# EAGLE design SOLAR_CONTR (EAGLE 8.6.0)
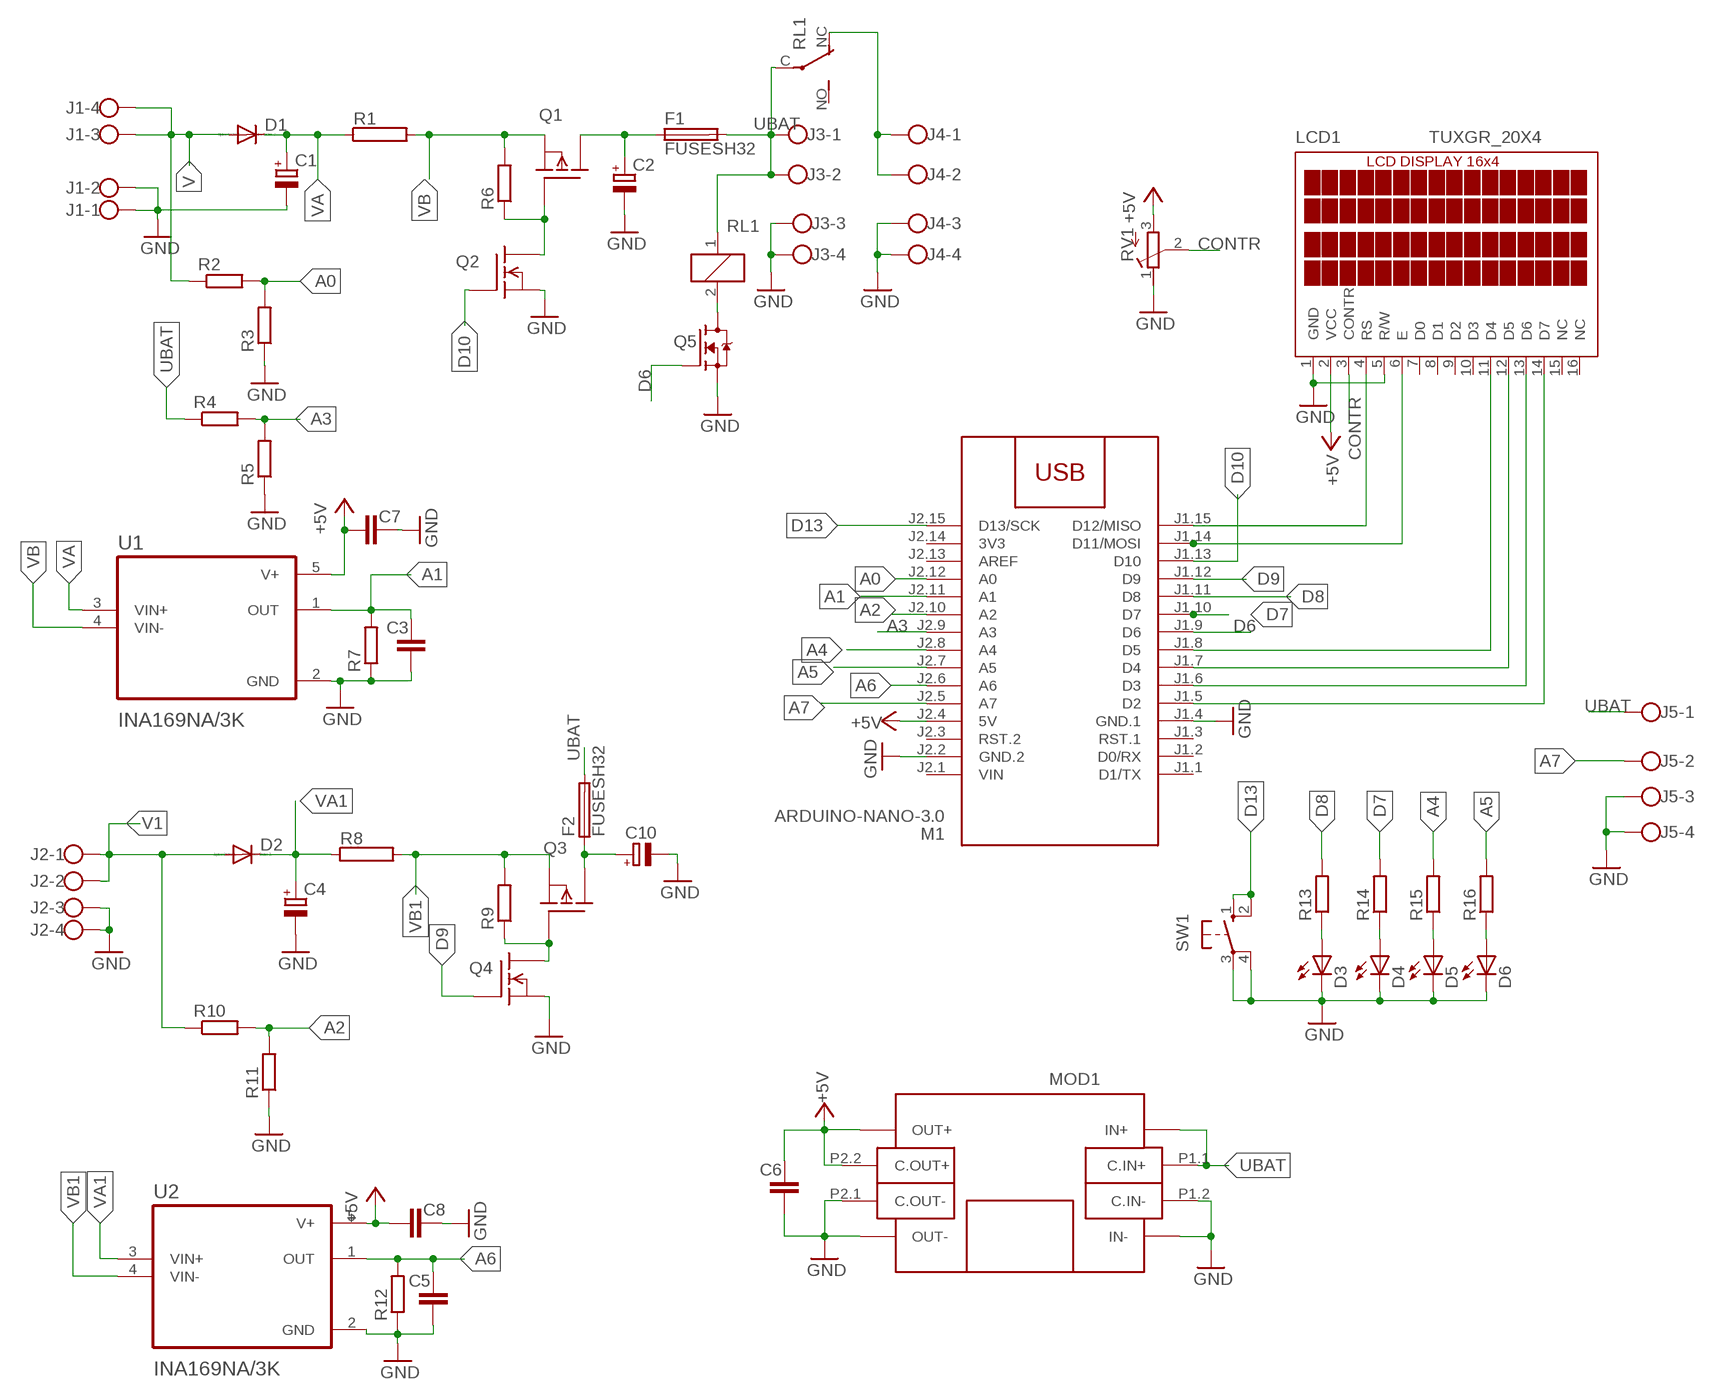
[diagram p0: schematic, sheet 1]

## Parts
C1  CPOL-EUE7.5-16  [E7,5-16]
C2  CPOL-EUE7.5-16  [E7,5-16]
C3  C-EUC1206  [C1206]
C4  CPOL-EUE7.5-16  [E7,5-16]
C5  C-EUC1206  [C1206]
C6  C-EUC1206  [C1206]
C7  C-EUC1206  [C1206]
C8  C-EUC1206  [C1206]
C10  CPOL-EUE7.5-16  [E7,5-16]
D1  BYT08P  [TO220ACS]
D2  BYT08P  [TO220ACS]
D3  LED5MM  [LED5MM]
D4  LED5MM  [LED5MM]
D5  LED5MM  [LED5MM]
D6  LED5MM  [LED5MM]
F1  FUSESH32  [SH32]
F2  FUSESH32  [SH32]
J1  W237-4  [W237-4]
J2  W237-4  [W237-4]
J3  W237-4  [W237-4]
J4  W237-4  [W237-4]
J5  W237-4  [W237-4]
LCD1  TUXGR_20X4  [TUXGR_20X4]
M1  ARDUINO-NANO-3.0  [ARDUINO-NANO-3.0]
MOD1  DC-DC-LM2596-DISP#RC  [DC-DC-LM2596-DISP#RC]
Q1  BUZ171  [TO220]
Q2  VN2222KM  [TO237]
Q3  BUZ171  [TO220]
Q4  VN2222KM  [TO237]
Q5  NTF3055L108  [SOT223]
R1  RAC05  [AC05]
R2  R-EU_R1206  [R1206]
R3  R-EU_R1206  [R1206]
R4  R-EU_R1206  [R1206]
R5  R-EU_R1206  [R1206]
R6  R-EU_R1206  [R1206]
R7  R-EU_R1206  [R1206]
R8  RAC05  [AC05]
R9  R-EU_R1206  [R1206]
R10  R-EU_R1206  [R1206]
R11  R-EU_R1206  [R1206]
R12  R-EU_R1206  [R1206]
R13  R-EU_R1206  [R1206]
R14  R-EU_R1206  [R1206]
R15  R-EU_R1206  [R1206]
R16  R-EU_R1206  [R1206]
RL1  JTN-PCB-DC9V  [JT-PCB]
RV1  R-TRIMM-3386-F  [R-TRIMM-3386F]
SW1  40-XX  [B3F-40XX]
U1  INA169NA/3K  [SOT95P280X145-5N]
U2  INA169NA/3K  [SOT95P280X145-5N]

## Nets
+5V: C6.1 C7.1 C8.1 LCD1.2(VCC) M1.J2.4(5V) MOD1.OUT+ MOD1.P2.2(C.OUT+) RV1.3(E) U1.5(V+) U2.5(V+)
A0: M1.J2.12(A0) R2.2 R3.2
A1: C3.1 M1.J2.11(A1) R7.2 U1.1(OUT)
A2: M1.J2.10(A2) R10.2 R11.2
A3: M1.J2.9(A3) R4.2 R5.2
A4: M1.J2.8(A4) R15.2
A5: M1.J2.7(A5) R16.2
A6: C5.1 M1.J2.6(A6) R12.2 U2.1(OUT)
A7: J5.2 M1.J2.5(A7)
CONTR: LCD1.3(CONTR) RV1.2(S)
D6: M1.J1.9(D6) Q5.1(G)
D7: M1.J1.10(D7) R14.2
D8: M1.J1.11(D8) R13.2
D9: M1.J1.12(D9) Q4.2(G)
D10: M1.J1.13(D10) Q2.2(G)
D13: M1.J2.15(D13/SCK) SW1.1(S) SW1.2(S1)
GND: C1.- C2.- C3.2 C4.- C5.2 C6.2 C7.2 C8.2 C10.- D3.K(C) D4.K(C) D5.K(C) D6.K(C) J1.1 J1.2 J2.3 J2.4 J3.3 J3.4 J4.3 J4.4 J5.3 J5.4 LCD1.1(GND) LCD1.5(R/W) M1.J1.4(GND.1) M1.J2.2(GND.2) MOD1.IN- MOD1.OUT- MOD1.P1.2(C.IN-) MOD1.P2.1(C.OUT-) Q2.3(S) Q4.3(S) Q5.3(S) R3.1 R5.1 R7.1 R11.1 R12.1 RV1.1(A) SW1.3(P) SW1.4(P1) U1.2(GND) U2.2(GND)
N$1: LCD1.4(RS) M1.J1.15(D12/MISO)
N$2: LCD1.6(E) M1.J1.14(D11/MOSI)
N$3: LCD1.11(D4) M1.J1.8(D5)
N$4: LCD1.12(D5) M1.J1.7(D4)
N$5: LCD1.13(D6) M1.J1.6(D3)
N$6: LCD1.14(D7) M1.J1.5(D2)
N$7: C2.+ F1.1A Q1.2(D)
N$8: Q5.2(D) Q5.4(D) RL1.2
N$9: Q1.1(G) Q2.1(D) R6.1
N$10: Q3.1(G) Q4.1(D) R9.1
N$11: C10.+ F2.1A Q3.2(D)
N$13: J4.1 J4.2 RL1.NC(O)
N$14: D3.A R13.1
N$15: D4.A R14.1
N$16: D5.A R15.1
N$17: D6.A R16.1
UBAT: F1.2A F2.2A J3.1 J3.2 J5.1 MOD1.IN+ MOD1.P1.1(C.IN+) R4.1 RL1.1 RL1.C(P)
V: D1.A J1.3 J1.4 R2.1
V1: D2.A J2.1 J2.2 R10.1
VA: C1.+ D1.C R1.1 U1.3(VIN+)
VA1: C4.+ D2.C R8.1 U2.3(VIN+)
VB: Q1.3(S) R1.2 R6.2 U1.4(VIN-)
VB1: Q3.3(S) R8.2 R9.2 U2.4(VIN-)
Unconnected: LCD1.7(D0) LCD1.8(D1) LCD1.9(D2) LCD1.10(D3) LCD1.15(NC) LCD1.16(NC) M1.J1.1(D1/TX) M1.J1.2(D0/RX) M1.J1.3(RST.1) M1.J2.3(RST.2) M1.J2.13(AREF) RL1.NO(S)

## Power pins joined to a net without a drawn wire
3V3: M1.J2.14(3V3)
VIN: M1.J2.1(VIN)

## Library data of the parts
C1 C2 C4 C10 = rcl:CPOL-EU: POLARIZED CAPACITOR, European symbol
C3 C5-C8 = rcl:C-EU: CAPACITOR, European symbol
D1 D2 = diode:BYT08P: DIODE
D3-D6 = led:LED: LED
F1 F2 = fuse:FUSE: Fuse; OC_FARNELL: unknown; OC_NEWARK: unknown
J1-J5 = con-wago-500:W237-4: WAGO SCREW CLAMP; OC_FARNELL: unknown; OC_NEWARK: unknown
LCD1 = display-lcd:TUXGR_20X4: LCD DISPLAY 20X4
M1 = diy-modules:ARDUINO-NANO-3.0: Arduino Nano 3.0 and compatible devices More details available here: https://www.arduino.cc/en/Main/ArduinoBoardNano Click here to find device on ebay.com
MOD1 = diy-modules:DC-DC-LM2596-DISP#RC: DC/DC Step-Down Regulator with Voltage Display based on LM2596-ADJ chip Symbol with input and output connectors More details available here: http://www.instructables.com/id/The-Introduction-of-LM2596-Step-Down-Power-Module-/ LM2596 datasheet available here: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
Q1 Q3 = transistor-fet:BUZ171: P-Channel Enhancement MOSFET -50V; 7A; 0,4Ohm
Q2 Q4 = transistor-fet:VN2222KM: N-Channel Enhancement MOSFET (VMOS); 60V; 0,5A; 7,5Ohm
Q5 = transistor-fet:NTF3055L108
R1 R8 = resistor-power:R: Power Resitor; OC_FARNELL: unknown; OC_NEWARK: unknown
R2-R7 R9-R16 = rcl:R-EU_: RESISTOR, European symbol
RL1 = relay:JT?-*: COMPACT ECONOMICAL 30 AMP. RELAY NAiS Source: http://www.mew-europe.com/.. en_ds_61212_0000.pdf; OC_FARNELL: unknown; OC_NEWARK: unknown
RV1 = rcl:R-TRIMM-3386-F
SW1 = switch-omron:40-XX: OMRON SWITCH; MF: OMRON COMPONENTS USA; MPN: B3F-4000; OC_FARNELL: 176434; OC_NEWARK: 36K3105
U1 U2 = INA169NA_3K:INA169NA/3K: Check availability; AVAILABILITY: In Stock; CHECK_PRICES: https://www.snapeda.com/parts/INA169NA/3K/Texas+Instruments/view-part/?ref=eda; DESCRIPTION: 2.7 to 60V, 440kHz Variable gain current sense amplifier; MF: Texas Instruments; MP: INA169NA/3K; PACKAGE: SOT-23-5 Texas Instruments; PRICE: None; PURCHASE-URL: https://pricing.snapeda.com/search?q=INA169NA/3K&ref=eda; SNAPEDA_LINK: https://www.snapeda.com/parts/INA169NA/3K/Texas+Instruments/view-part/?ref=snap

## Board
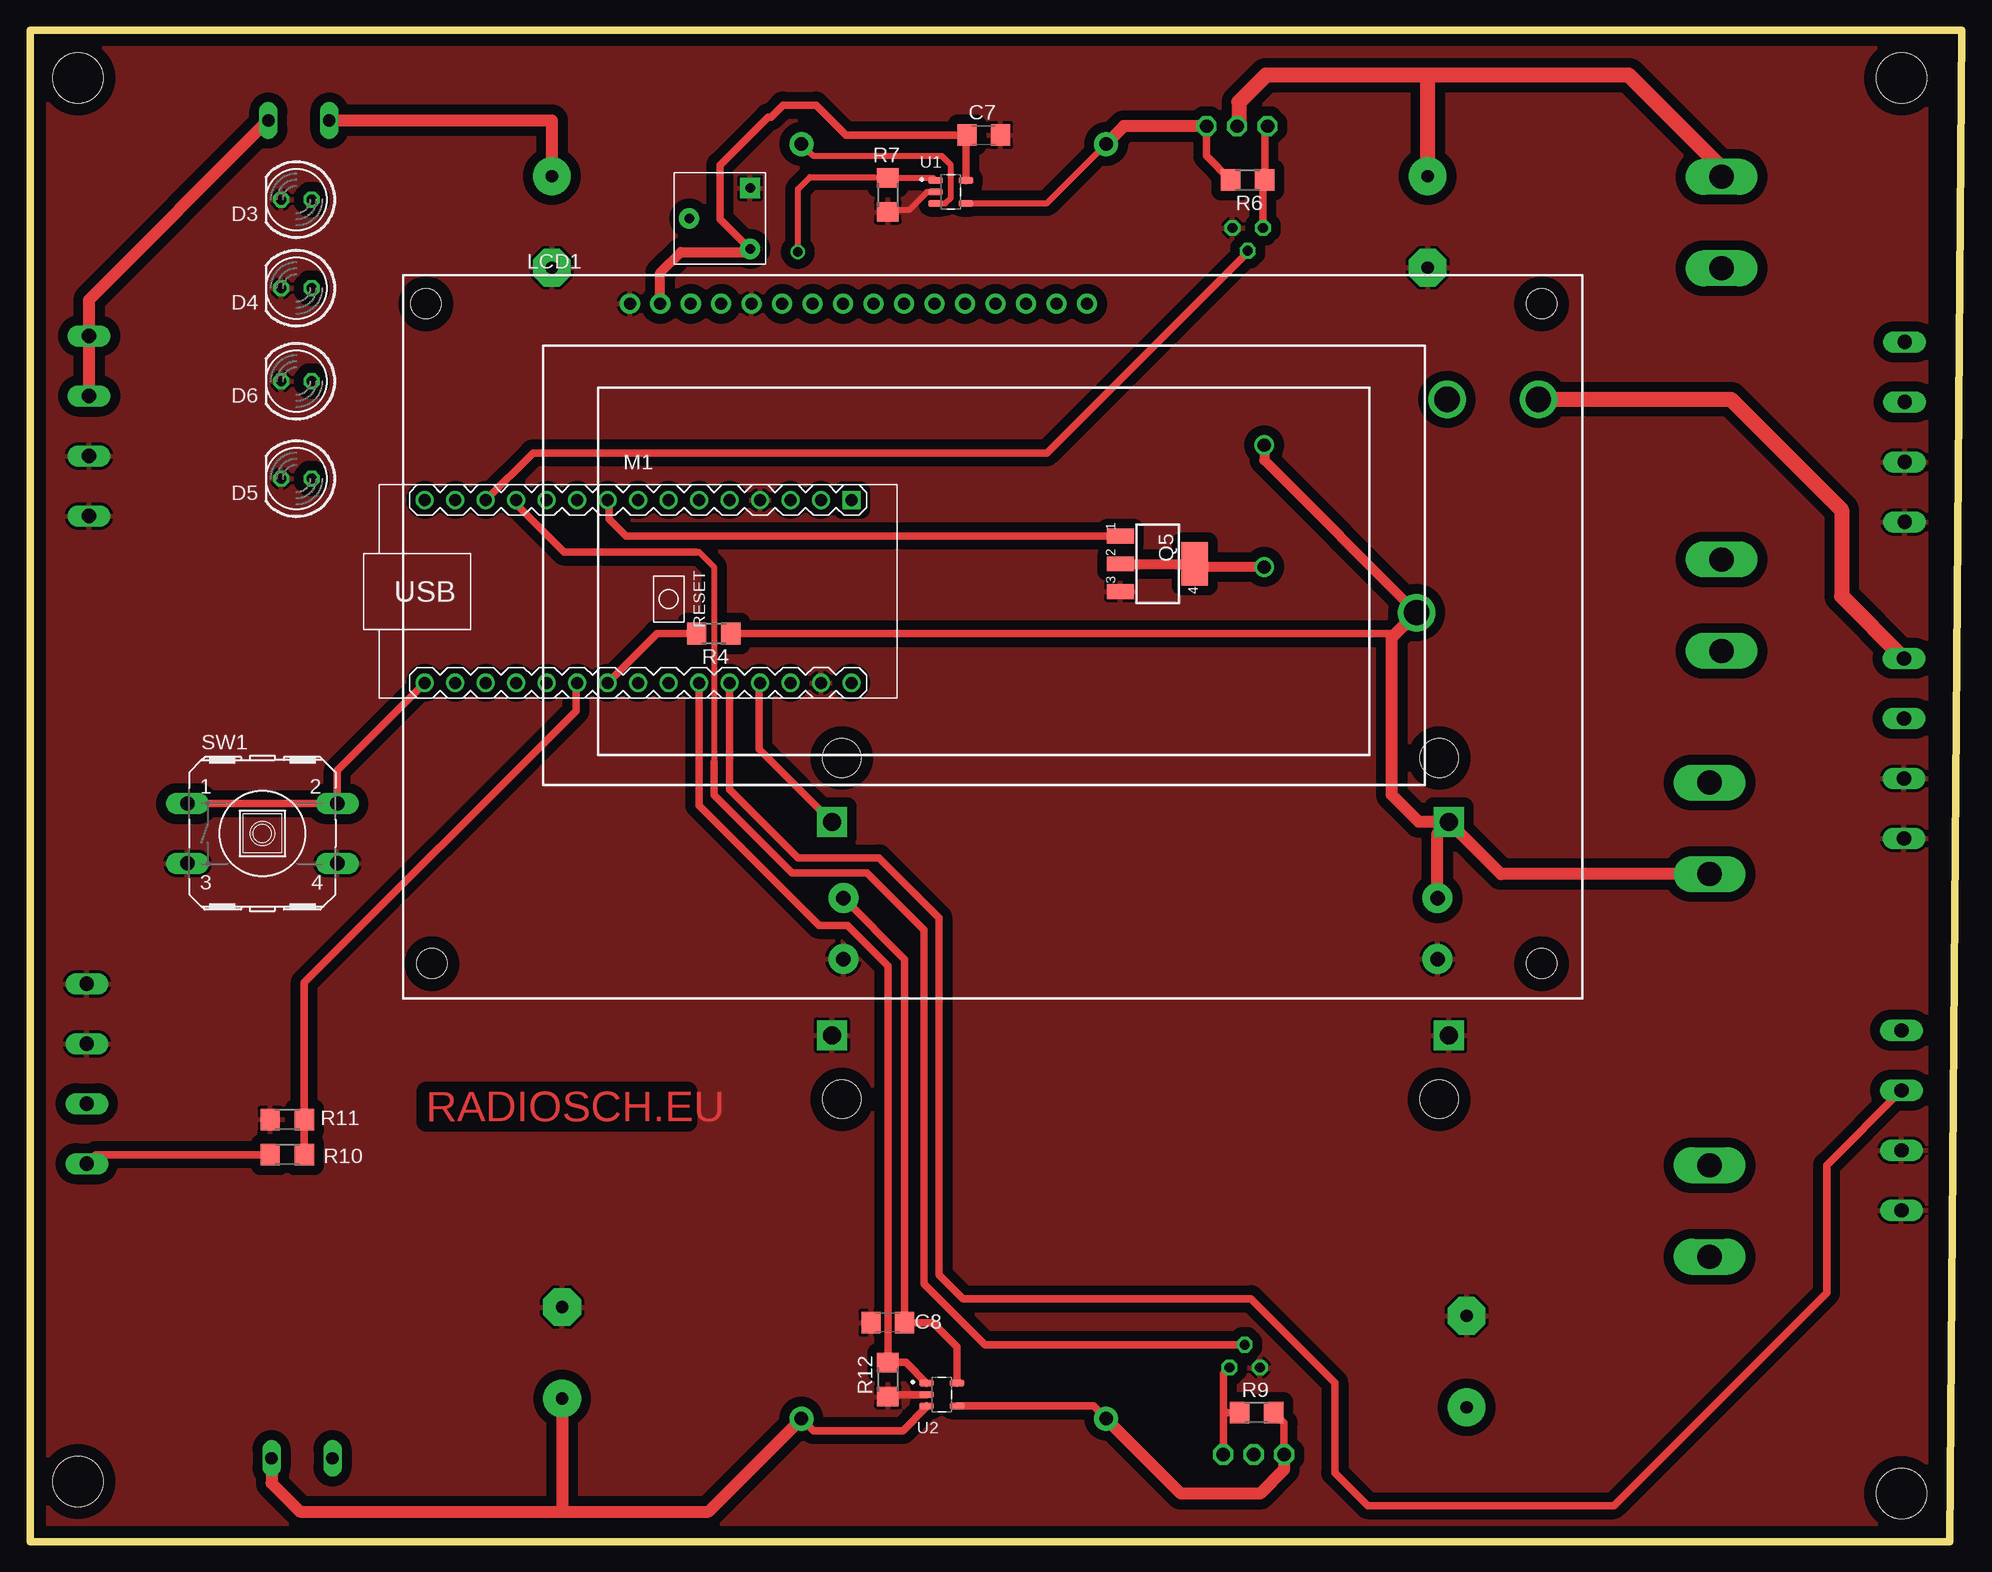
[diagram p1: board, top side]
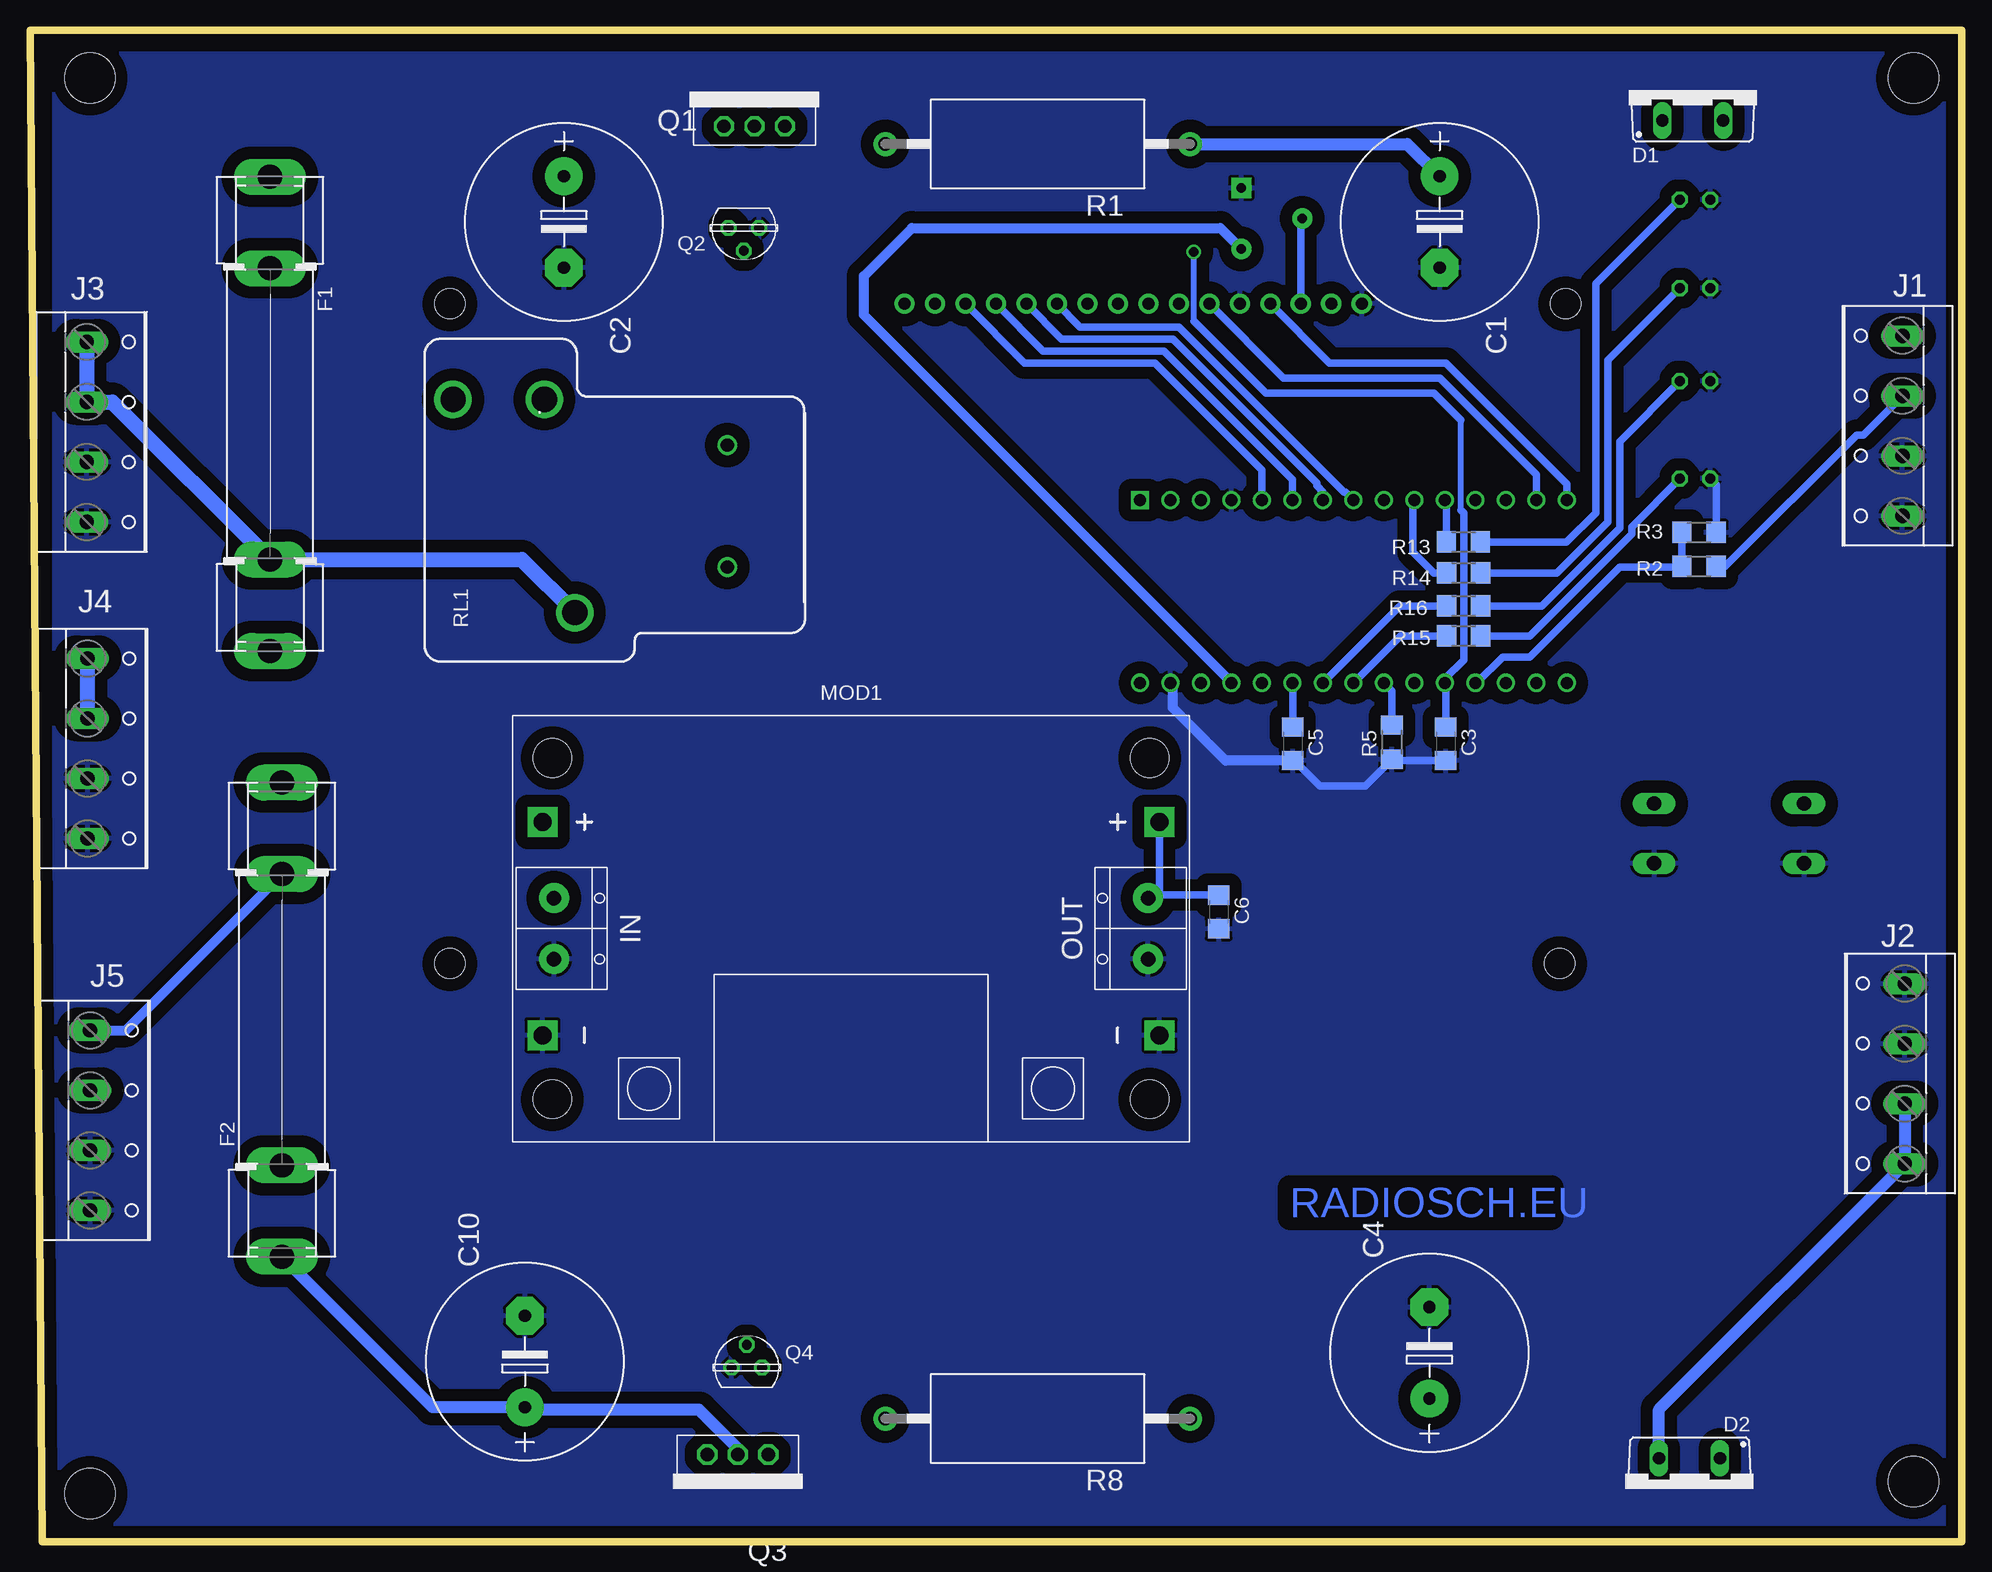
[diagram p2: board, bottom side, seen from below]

Size 161 x 126 mm. Coordinates in mm from the lower left corner, seen from the top.
Outline: 0,0 160,0 161,126 0,126 0,0
Copper layers (1*16): Top 0.035mm / dielectric 1.5mm / Bottom 0.035mm
Design rules "default": minimum track width 10mil, minimum drill 24mil, track to track 8mil, track to pad 8mil, pad to pad 8mil, via to via 8mil, smd to smd 8mil, copper to edge 40mil, drill to drill 8mil, minimum pad ring 10mil, minimum via ring 8mil, stop-mask expansion 4mil, vias tented up to drill 0mil, thermal gap 10mil
Holes 4.2 mm at 4,122 4,5 156,4 156,122

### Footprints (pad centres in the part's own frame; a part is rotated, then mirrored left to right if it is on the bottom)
E7,5-16 = drill 1.016 pad 3.15: + -3.81,0 | drill 1.016 pad 3.15 octagon: - 3.81,0
C1206 = smd 1.6 x 1.8: 1 -1.4,0; 2 1.4,0
TO220ACS = drill 1.016 long: A 2.54,-2.54; C -2.54,-2.54
LED5MM = drill 0.813 octagon: A -1.27,0; K 1.27,0
SH32 = drill 2.007 long: 1A -16.764,0; 1B -9.144,0; 2A 15.144,0; 2B 22.764,0
W237-4 = drill 1.194 long: 1 -7.5,-1.27; 2 -2.5,-1.27; 3 2.5,-1.27; 4 7.5,-1.27
TUXGR_20X4 = drill 1 pad 1.676: 1 11.14,-2.28; 2 13.68,-2.28; 3 16.22,-2.28; 4 18.76,-2.28; 5 21.3,-2.28; 6 23.84,-2.28; 7 26.38,-2.28; 8 28.92,-2.28; 9 31.46,-2.28; 10 34,-2.28; 11 36.54,-2.28; 12 39.08,-2.28; 13 41.62,-2.28; 14 44.16,-2.28; 15 46.7,-2.28; 16 49.24,-2.28 | hole 2.5: -5.36,-57.28; 87.14,-57.28; -5.86,-2.28; 87.14,-2.28
ARDUINO-NANO-3.0 = drill 1 square: J1.1 17.78,7.62 | drill 1: J1.2 15.24,7.62; J1.3 12.7,7.62; J1.4 10.16,7.62; J1.5 7.62,7.62; J1.6 5.08,7.62; J1.7 2.54,7.62; J1.8 0,7.62; J1.9 -2.54,7.62; J1.10 -5.08,7.62; J1.11 -7.62,7.62; J1.12 -10.16,7.62; J1.13 -12.7,7.62; J1.14 -15.24,7.62; J1.15 -17.78,7.62; J2.1 17.78,-7.62; J2.2 15.24,-7.62; J2.3 12.7,-7.62; J2.4 10.16,-7.62; J2.5 7.62,-7.62; J2.6 5.08,-7.62; J2.7 2.54,-7.62; J2.8 0,-7.62; J2.9 -2.54,-7.62; J2.10 -5.08,-7.62; J2.11 -7.62,-7.62; J2.12 -10.16,-7.62; J2.13 -12.7,-7.62; J2.14 -15.24,-7.62; J2.15 -17.78,-7.62
DC-DC-LM2596-DISP#RC = drill 1.5 pad 2.5 square: IN+ -25.718,8.89; IN- -25.718,-8.89; OUT+ 25.718,8.89; OUT- 25.718,-8.89 | drill 1.2 pad 2.5: P1.1 -24.765,2.54; P1.2 -24.765,-2.54; P2.1 24.765,-2.54; P2.2 24.765,2.54 | hole 3.2: -24.892,14.224; 24.892,-14.224; 24.892,14.224; -24.892,-14.224
TO220 = drill 1.118 octagon: 1 -2.54,0; 2 0,0; 3 2.54,0
TO237 = drill 0.813 octagon: 1 1.27,0; 2 0,1.905; 3 -1.27,0
SOT223 = smd 1.219 x 2.235: 1 -2.311,-3.099; 2 0,-3.099; 3 2.311,-3.099 | smd 3.6 x 2.2: 4 0,3.099
AC05 = drill 1.1 pad 2: 1 -12.7,0; 2 12.7,0
R1206 = smd 1.6 x 1.803: 1 -1.422,0; 2 1.422,0
JT-PCB = drill 1.1: 1 5.08,0; 2 -5.08,0 | drill 2.1: C -8.89,12.7; NC 8.89,22.86; NO 8.89,15.24
R-TRIMM-3386F = drill 0.8 pad 1.676 square: 1 0,0 | drill 0.8 pad 1.676: 2 5.08,2.54; 3 0,5.08
B3F-40XX = drill 1.194 long: 1 -6.248,2.489; 2 6.248,2.489; 3 -6.248,-2.489; 4 6.248,-2.489
SOT95P280X145-5N = smd 1.21 x 0.59: 1 -1.255,0.95; 2 -1.255,0; 3 -1.255,-0.95; 4 1.255,-0.95; 5 1.255,0.95

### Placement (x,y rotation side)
C1  43.5,110 270 bottom
C2  116.5,110 270 bottom
C3  43,66.5 270 bottom
C4  44.35,15.73 90 bottom
C5  55.75,66.5 270 bottom
C6  61.91,52.48 270 bottom
C7  79.5,117.25 0 top
C8  71.5,18.25 180 top
C10  119.75,15 90 bottom
D1  22.41,121 0 bottom
D2  22.67,4.39 180 bottom
D3  22.21,111.86 180 top
D4  22.21,104.48 180 top
D5  22.21,88.6 180 top
D6  22.21,96.72 180 top
F1  141,97 270 bottom
F2  140,40.5 90 bottom
J1  6.2,93 90 bottom
J2  6,39 90 bottom
J3  155,92.5 270 bottom
J4  154.93,66.11 270 bottom
J5  154.72,35.11 270 bottom
LCD1  38.86,105.46 0 top
M1  50.69,79.2 0 top
MOD1  92.56,51.09 0 bottom
Q1  100.61,117.98 0 bottom
Q2  101.5,109.5 180 bottom
Q3  102,7.25 180 bottom
Q4  101.25,14.5 0 bottom
Q5  94,81.5 270 top
R1  77,116.5 180 bottom
R2  21.88,81.28 180 bottom
R3  21.88,84.11 180 bottom
R4  56.99,75.69 180 top
R5  47.48,66.63 90 bottom
R6  101.5,113.5 180 top
R7  71.5,112.25 90 top
R8  77,10.25 180 bottom
R9  102.25,10.75 0 top
R10  21.45,32.25 0 top
R11  21.45,35.17 0 top
R12  71.5,13.5 90 top
R13  41.52,83.32 180 bottom
R14  41.5,80.75 180 bottom
R15  41.5,75.5 180 bottom
R16  41.5,78 180 bottom
RL1  102.88,86.32 90 bottom
RV1  60.03,112.83 180 top
SW1  19.37,59.03 0 top
U1  76.75,112.5 0 top
U2  76,12.25 0 top

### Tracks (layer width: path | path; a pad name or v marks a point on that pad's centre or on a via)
+5V
  Top 0.61: RV1.3 60,107.75 57.5,110.25 57.5,114.75 61.5,118.75 61.75,118.75 62.75,119.75 65.5,119.75 68,117.25 C7.1 78,117.16 U1.5 | M1.J2.4 60.75,71.48 60.75,66.07 MOD1.OUT+ | MOD1.P2.2 72.9,48.52 C8.1 75.25,18.25 77.25,16.25 U2.5
  Top 0.813: LCD1.2 52.54,105.79 54.25,107.5 59.78,107.5 RV1.3
  Bottom 0.61: C6.1 67.25,53.88 | 67.25,53.88 67.55,53.88 MOD1.P2.2 | MOD1.OUT+ 66.84,54.29 67.25,53.88
  Bottom 0.813: M1.J2.4 60.85,71.6 91.5,102.25 91.5,105.5 87.5,109.5 61.78,109.5 RV1.3
A0
  Bottom 0.61: M1.J2.12 40.42,71.58 38.25,73.75 36,73.75 28.5,81.25 23.33,81.25 R2.2 R3.2
A1  (via drill 0.8)
  Top 0.51: U1.1 75.27,113.67 R7.2 71.42,113.75 65,113.75 64,112.75 v64,107.5
  Bottom 0.5: 41.75,86 41.75,93.5 | 64,101.75 v64,107.5
  Bottom 0.61: C3.1 43,71.51 M1.J2.11 43.07,71.93 41.5,73.5 41.5,85.75 41.75,86 | 41.75,93.5 44,95.75 58,95.75 64,101.75
A2
  Top 0.61: R10.2 R11.2 22.87,46.62 45.5,69.25 45.5,71.47 M1.J2.10
A3
  Top 0.61: R4.2 52.26,75.69 M1.J2.9
  Bottom 0.61: R5.2 47.48,70.91 M1.J2.9
A4
  Bottom 0.61: R15.2 46.77,75.5 M1.J2.8
A5
  Bottom 0.61: R16.2 46.81,78 M1.J2.7
A6
  Top 0.61: M1.J2.6 55.75,71.56 55.75,61.38 65.75,51.38 68.12,51.38 71.5,48 R12.2 73.02,14.92 U2.1
  Bottom 0.61: C5.1 55.75,71.56 M1.J2.6
A7
  Top 0.61: M1.J2.5 58.31,62.69 64,57 70.75,57 75.75,52 75.75,22.25 77.75,20.25 101.75,20.25 108.75,13.25 108.75,5.75 111.5,3 132,3 149.75,20.75 149.75,31.37 J5.2
CONTR
  Bottom 0.61: LCD1.3 55.08,110.16 RV1.2
D6
  Top 0.61: Q5.1 49.69,83.81 48.25,85.25 48.25,86.72 M1.J1.9
D7
  Bottom 0.61: R14.2 44,80.75 45.75,82.5 45.75,86.68 M1.J1.10
D8
  Bottom 0.61: R13.2 42.94,86.69 M1.J1.11
D9
  Top 0.51: 55.5,82.5 55.75,82.5 57,81.25 57,65
  Top 0.61: M1.J1.12 40.53,86.47 44.5,82.5 55.5,82.5 | 57,65 57,62.25 63.5,55.75 69.75,55.75 74.5,51 74.5,21.5 79.59,16.41 Q4.2
D10
  Top 0.61: Q2.2 101.5,107.5 84.75,90.75 41.92,90.75 M1.J1.13
D13
  Top 0.61: SW1.1 SW1.2 25.62,64.29 M1.J2.15
GND
  Top 0.51: U1.2 74.75,112.5 73.25,111 71.67,111 R7.1
  Top 0.61: U2.2 71.67,12.25 R12.1
  Bottom 0.61: C3.2 47.37,65.1 R5.1 49.69,63 53.5,63 55.6,65.1 C5.2 | R3.1 20.46,88.12 D5.K
  Bottom 0.813: C5.2 61.35,65.1 65.75,69.5 65.75,71.4 M1.J2.2
  pour Top (isolate 0.813): 1,125 158,125 158,1 1,1
  pour Bottom (isolate 1.016): 159,124 159,1 0.75,1 0.75,124
N$1
  Bottom 0.61: M1.J1.15 32.91,88.16 43,98.25 52.69,98.25 LCD1.4
N$2
  Bottom 0.61: M1.J1.14 35.45,88.95 43.5,97 56.52,97 LCD1.6
N$3
  Bottom 0.61: LCD1.11 73.47,101.25 65.25,101.25 51.5,87.5 51.37,87.5 M1.J1.8
N$4
  Bottom 0.61: M1.J1.7 53.23,87.5 53.75,88.02 53.75,88.25 65.75,100.25 75.01,100.25 LCD1.12
N$5
  Bottom 0.61: M1.J1.6 55.77,88.52 66.5,99.25 76.55,99.25 LCD1.13
N$6
  Bottom 0.61: M1.J1.5 58.31,89.31 67.25,98.25 78.09,98.25 LCD1.14
N$7
  Top 1.27: F1.1A 141,114.5 133.25,122.25 116.5,122.25 | 116.5,122.25 103,122.25 100.75,120 100.75,118.12 Q1.2 | C2.+ 116.5,122.25
N$8
  Top 0.813: Q5.2 96.5,81.5 | 96.5,81.5 Q5.4 | RL1.2 96.76,81.24 96.5,81.5
N$9
  Top 0.61: Q1.1 102.92,117.75 R6.1 102.77,113.35 Q2.1
N$10
  Top 0.61: Q3.1 99.46,11 | 99.46,11 99.46,13.98 Q4.1 | R9.1 99.71,10.75 99.46,11
N$11
  Bottom 1.016: Q3.2 102,7.75 105.25,11 119.56,11 C10.+ 127.45,11.19 F2.1A
N$13
  Top 1.27: RL1.NC 141.79,95.21 151,86 151,78.81 J4.1
  Bottom 1.27: J4.2 J4.1
N$14
  Bottom 0.61: R13.1 32.93,83.32 30.5,85.75 30.5,104.84 D3.A
N$15
  Bottom 0.61: R14.1 33.75,80.75 29.5,85 29.5,98.46 D4.A
N$16
  Bottom 0.61: R15.1 36,75.5 27.5,84 27.5,84.58 D5.A
N$17
  Bottom 0.61: R16.1 35,78 28.5,84.5 28.5,91.7 D6.A
UBAT
  Top 0.61: R4.1 113.84,75.69 RL1.C
  Top 0.813: RL1.1 102.88,90.13 RL1.C
  Top 1.016: MOD1.IN+ 115.77,59.98 113.5,62.25 113.5,75.35 RL1.C | MOD1.P1.1 117.33,59.03 MOD1.IN+ | F2.2A 122.61,55.64 MOD1.IN+
  Bottom 0.813: J5.1 153.03,42.61 F2.2A
  Bottom 1.27: 115.75,77.26 RL1.C 120.01,81.86 F1.2A 154.14,95 J3.2 J3.1
V
  Top 1.016: J1.3 J1.4 4.93,103.52 D1.A
  Bottom 0.61: R2.1 19.72,81.28 8.75,92.25 8.18,92.25 J1.3
V1
  Top 0.61: R10.1 5.48,32.25 J2.1
  Bottom 1.016: D2.A 25.21,11.02 J2.1 J2.2
VA
  Top 0.51: U1.3 76.3,111.55 76.75,112 76.75,114.75 76,115.5 65.3,115.5 R1.1
  Top 1.016: D1.C 43.5,118.46 C1.+
  Bottom 1.016: R1.1 46.19,116.5 C1.+
VA1
  Top 0.61: U2.3 74.75,11.24 72.75,9.25 65.3,9.25 R8.1
  Top 1.016: D2.C 20.13,4.87 22.5,2.5 44.25,2.5 | 44.25,2.5 56.55,2.5 R8.1 | C4.+ 44.35,2.6 44.25,2.5
VB
  Top 0.51: U1.4 84.75,111.55 R1.2
  Top 0.61: Q1.3 98.07,115.51 R6.2
  Top 1.016: Q1.3 91.18,117.98 R1.2
VB1
  Top 0.61: U2.4 88.65,11.3 R8.2 | Q3.3 104.54,9.88 R9.2
  Top 1.016: Q3.3 104.54,6.04 102.5,4 95.95,4 R8.2

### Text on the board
Top: RADIOSCH.EU
Bottom: RADIOSCH.EU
